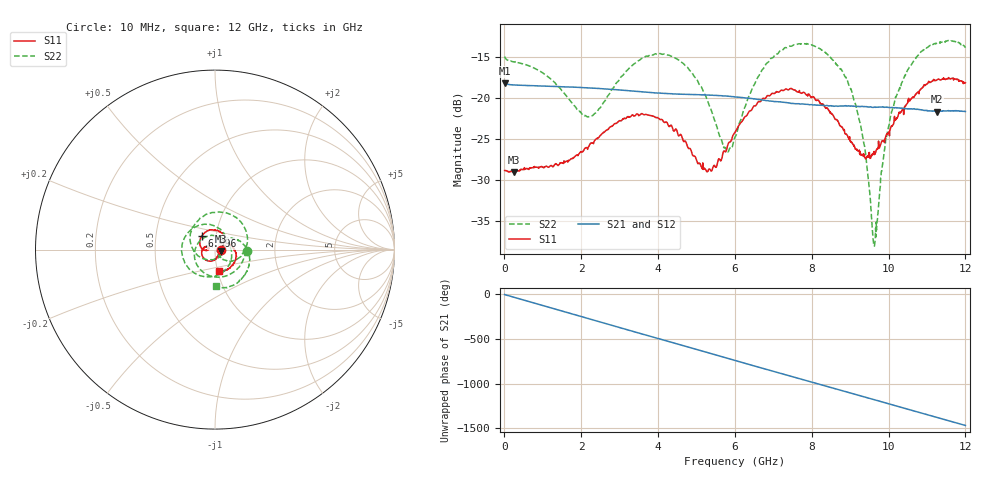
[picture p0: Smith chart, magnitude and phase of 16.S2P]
!Agilent Technologies,E5071C,MY46316741,A.11.02
!Date: Wed Sep 16 11:45:14 2020
!Data & Calibration Information:
!Freq	S11:SOLT2(ON)	S21:SOLT2(ON)	S12:SOLT2(ON)	S22:SOLT2(ON)
!PortZ  Port1:50+j0  Port2:50+j0
!Above PortZ is port z conversion or system Z0 setting when saving the data.
!When reading, reference impedance value at option line is always used.
# Hz S dB R 50
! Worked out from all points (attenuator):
!   1561 points, 10 MHz to 12 GHz, reference 50 ohm
!   highest |S21| = -18.21 dB at 10 MHz (marker M1); lowest = -21.7 dB at 11.27 GHz (marker M2)
!   lowest |S11| = -29.1 dB at 255.9 MHz (marker M3), VSWR 1.07, Z = 53.5 - j0.789 ohm
!   |S11| at or under -10 dB: start of sweep to end of sweep
!   |S22| runs from -38.1 to -13.0 dB; largest |S21 - S12| = 0.001
!   S11 on the Smith chart (normalised r, x): 10 MHz: 1.07, -0.00; 6.996 GHz: 0.85, +0.13; 12 GHz: 1.02, -0.25
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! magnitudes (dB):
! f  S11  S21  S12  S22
! 10 MHz  -28.9  -18.2  -18.2  -14.9
! 255.9 MHz  -29.1  -18.4  -18.4  -15.6
! 1.132 GHz  -28.5  -18.6  -18.6  -17.4
! 2.016 GHz  -26.6  -18.7  -18.7  -21.9
! 2.37 GHz  -25.1  -18.8  -18.8  -21.9
! 3.161 GHz  -22.5  -19.1  -19.1  -16.8
! 4.007 GHz  -22.5  -19.4  -19.4  -14.7
! 4.691 GHz  -25.3  -19.6  -19.6  -15.9
! 5.267 GHz  -29.0  -19.7  -19.7  -20.0
! 5.759 GHz  -26.6  -19.8  -19.8  -26.2
! 6.005 GHz  -24.2  -19.9  -19.9  -24.8
! 6.466 GHz  -21.2  -20.1  -20.1  -18.7
! 6.996 GHz  -19.5  -20.4  -20.4  -15.1
! 8.011 GHz  -19.9  -20.8  -20.9  -13.5
! 8.757 GHz  -23.5  -21.0  -21.0  -16.5
! 9.056 GHz  -25.6  -21.0  -21.0  -19.5
! 9.379 GHz  -27.3  -21.1  -21.1  -26.0
! 9.617 GHz  -26.7  -21.2  -21.1  -38.0
! 10 GHz  -24.3  -21.2  -21.2  -23.5
! 10.51 GHz  -20.2  -21.3  -21.4  -16.5
! 11.27 GHz  -17.8  -21.7  -21.6  -13.3
! 12 GHz  -18.2  -21.7  -21.7  -13.9
